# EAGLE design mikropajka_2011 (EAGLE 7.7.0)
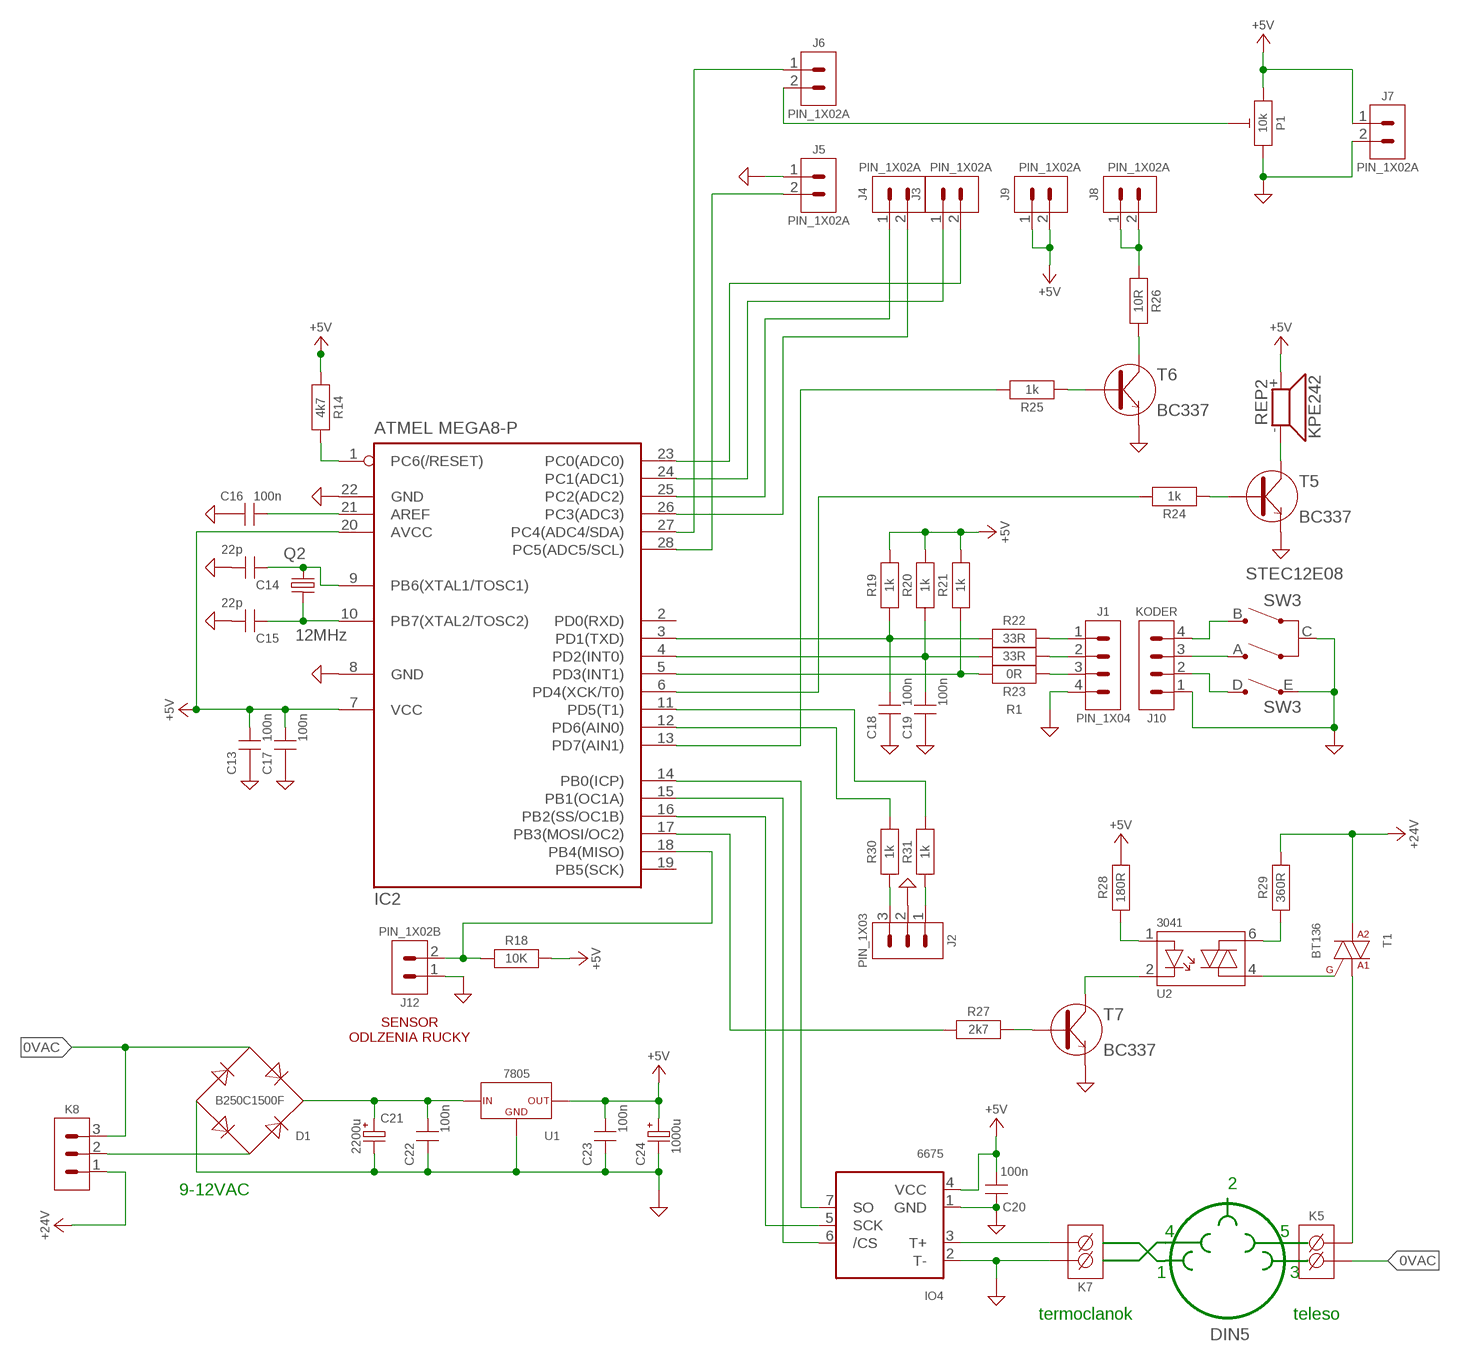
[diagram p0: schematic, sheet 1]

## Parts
C13  100n  KERAMICKYA  [CK_5.08/A]
C14  22p  KERAMICKYB  [CK_5.08/B]
C15  22p  KERAMICKYB  [CK_5.08/B]
C16  100n  KERAMICKYA  [CK_5.08/A]
C17  100n  KERAMICKYA  [CK_5.08/A]
C18  100n  KERAMICKYA  [CK_5.08/A]
C19  100n  KERAMICKYA  [CK_5.08/A]
C20  100n  KERAMICKYA  [CK_5.08/A]
C21  2200u  ELEKTROLYTICKYD  [CE_7.5/A]
C22  100n  KERAMICKYA  [CK_5.08/A]
C23  100n  KERAMICKYA  [CK_5.08/A]
C24  1000u  ELEKTROLYTICKYC  [CE_5.08/B]
D1  B250C1500F  USMERNOVACI_MOSTIKA  [D.USMERNOVAC/GULATY]
IC2  ATMEL MEGA8-P  MEGA8-P  [DIL28-3]
IO4  6675  MAX6675  [SO08]
J1  PIN_1X04  [1X04]
J2  PIN_1X03  [1X03]
J3  PIN_1X02A  [1X02/A]
J4  PIN_1X02A  [1X02/A]
J5  PIN_1X02A  [1X02/A]
J6  PIN_1X02A  [1X02/A]
J7  PIN_1X02A  [1X02/A]
J8  PIN_1X02A  [1X02/A]
J9  PIN_1X02A  [1X02/A]
J10  KODER  PIN_1X04  [1X04]
J12  PIN_1X02B  [1X02/B]
K5  AKZ692/2  [AKZ692/2]
K7  AKZ692/2  [AKZ692/2]
K8  PSH02/3A  [PSH02/3A]
P1  10k  TRIMERE  [CA6]
Q2  12MHz  XTAL  [HC-49/U]
R1  0R  REZISTORA  [0207_10]
R14  4k7  REZISTORA  [0207_10]
R18  10K  REZISTOR  [0207_STOJATY]
R19  1k  REZISTORA  [0207_10]
R20  1k  REZISTORA  [0207_10]
R21  1k  REZISTORA  [0207_10]
R22  33R  REZISTORA  [0207_10]
R23  33R  REZISTORA  [0207_10]
R24  1k  REZISTORA  [0207_10]
R25  1k  REZISTORA  [0207_10]
R26  10R  REZISTORA  [0207_10]
R27  2k7  REZISTORA  [0207_10]
R28  180R  REZISTORA  [0207_10]
R29  360R  REZISTORA  [0207_10]
R30  1k  REZISTORA  [0207_10]
R31  1k  REZISTORA  [0207_10]
REP2  KPE242  [KPE242]
SW3  STEC12E08  KODER_ROTACNIEC12  [EC12]
T1  BT136  [TO220]
T5  BC337  [TO-92]
T6  BC337  [TO-92]
T7  BC337  [TO-92]
U1  7805  78..  [TO220]
U2  3041  MOC3041  [DIL6]

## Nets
0VAC: D1.AC+ K5.1 K8.3
24VAC: K8.1 R29.2 T1.2(A2) ; supply symbol labelled +24V
+5V: C13.C1 C17.C1 C20.C1 C23.C1 C24.C+ IC2.7(VCC) IC2.20(AVCC) IO4.4(VCC) J7.1 J9.1 J9.2 P1.3 R14.1 R18.2 R19.2 R20.2 R21.2 R28.2 REP2.+ U1.P3(OUT)
GND: C13.C2 C14.C1 C15.C1 C16.C2 C17.C2 C18.C2 C19.C2 C20.C2 C21.C- C22.C2 C23.C2 C24.C- D1.DC- IC2.8(GND) IC2.22(GND) IO4.1(GND) IO4.2(T-) J1.4 J2.2 J5.1 J7.2 J10.1 J12.1 K7.2 P1.1 SW3.C(A:C) SW3.E(B:E) T5.3(E) T6.3(E) T7.3(E) U1.P2(GND)
N$1: IC2.27(PC4(ADC4/SDA)) J6.1
N$2: J6.2 P1.2
N$3: J1.3 R1.1
N$4: C15.C2 IC2.10(PB7(XTAL2/TOSC2)) Q2.1
N$11: J8.1 J8.2 R26.1
N$41: C14.C2 IC2.9(PB6(XTAL1/TOSC1)) Q2.2
N$42: C16.C1 IC2.21(AREF)
N$43: IC2.1(PC6(/RESET)) R14.2
N$45: IC2.18(PB4(MISO)) J12.2 R18.1
N$48: R26.2 T6.1(C)
N$49: C18.C1 IC2.3(PD1(TXD)) R19.1 R22.2
N$50: C19.C1 IC2.4(PD2(INT0)) R20.1 R23.2
N$51: IC2.5(PD3(INT1)) R1.2 R21.1
N$52: J1.1 R22.1
N$53: J1.2 R23.1
N$54: IC2.13(PD7(AIN1)) R25.2
N$55: R24.1 T5.2(B)
N$56: IC2.6(PD4(XCK/T0)) R24.2
N$57: REP2.- T5.1(C)
N$58: IC2.17(PB3(MOSI/OC2)) R27.1
N$59: R25.1 T6.2(B)
N$60: R27.2 T7.2(B)
N$61: T7.1(C) U2.2
N$62: R28.1 U2.1
N$63: R29.1 U2.6
N$64: T1.3(G) U2.4
N$66: K5.2 T1.1(A1)
N$68: J2.3 R30.1
N$69: J2.1 R31.1
N$70: IC2.12(PD6(AIN0)) R30.2
N$71: IC2.11(PD5(T1)) R31.2
N$73: IO4.3(T+) K7.1
N$74: J10.4 SW3.B(A:B)
N$75: J10.3 SW3.A(A:A)
N$76: IC2.14(PB0(ICP)) IO4.7(SO)
N$77: IC2.15(PB1(OC1A)) IO4.6(/CS)
N$78: IC2.16(PB2(SS/OC1B)) IO4.5(SCK)
N$79: J10.2 SW3.D(B:D)
N$85: IC2.28(PC5(ADC5/SCL)) J5.2
N$87: IC2.23(PC0(ADC0)) J3.2
N$88: IC2.24(PC1(ADC1)) J3.1
N$89: IC2.25(PC2(ADC2)) J4.1
N$90: IC2.26(PC3(ADC3)) J4.2
N$91: C21.C+ C22.C1 D1.DC+ U1.P1(IN)
N$94: D1.AC- K8.2
Unconnected: IC2.2(PD0(RXD)) IC2.19(PB5(SCK))

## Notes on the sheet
- SENSOR
  ODLZENIA RUCKY
- 9-12VAC | 2
- 4 | 5
- 1 | 3
- termoclanok | teleso
- DIN5

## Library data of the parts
C13-C20 C22 C23 = Kondenzatory:KERAMICKY: Keramicky kondenzator
C21 C24 = Kondenzatory:ELEKTROLYTICKY: Elektrolyticky kondenzator
D1 = Diody:USMERNOVACI_MOSTIK: Usmeronovaci mostik
IC2 = atmel:MEGA8-P: MICROCONTROLLER 8 Kbytes FLASH, 1 kbytes SRAM, 512 bytes EEPROM, USART, 4-channel 10 bit ADC, 2-channel 8 bit ADC Pin compatible with Atmega48, ATMega88, ATMega168 Source: avr.lbr; OC_FARNELL: unknown; OC_NEWARK: unknown
IO4 = #PaJa_31:MAX6675: Cold Junction compensated K-Thermocouple to digital converter (0°C to + 1024°C)
J1 J10 = Pin:PIN_1X04: PIN_1x04
J2 = Pin:PIN_1X03: PIN_1x03
J3-J9 J12 = Pin:PIN_1X02: PIN_1x02
K5 K7 = Konektory:AKZ692/2: Svorkovnica 2 PIN
K8 = Konektory:PSH02/3: Konektor molex 3 PIN
P1 = Rezistory:TRIMER: Trimer
Q2 = Rozne:XTAL: Krystal
R1 R14 R18-R31 = Rezistory:REZISTOR: Rezistor 0207
REP2 = #PaJa_31:KPE242: Piezo-sirenka - 70dB - 3V az 16V
SW3 = #PaJa_22:KODER_ROTACNI: Rotacni koder se spinacem v hrideli www.tme.cz
T1 = Triak:BT136: BT136
T5-T7 = #PaJa_30:BC337: Tranzistor NPN - Univerzalni NF - Ic=0,5A
U1 = Stabilizatory:78..: Linearny stabilizator napatia 78.. (pozitivny)
U2 = Optotriak:MOC3041: Optotriak MOC3041

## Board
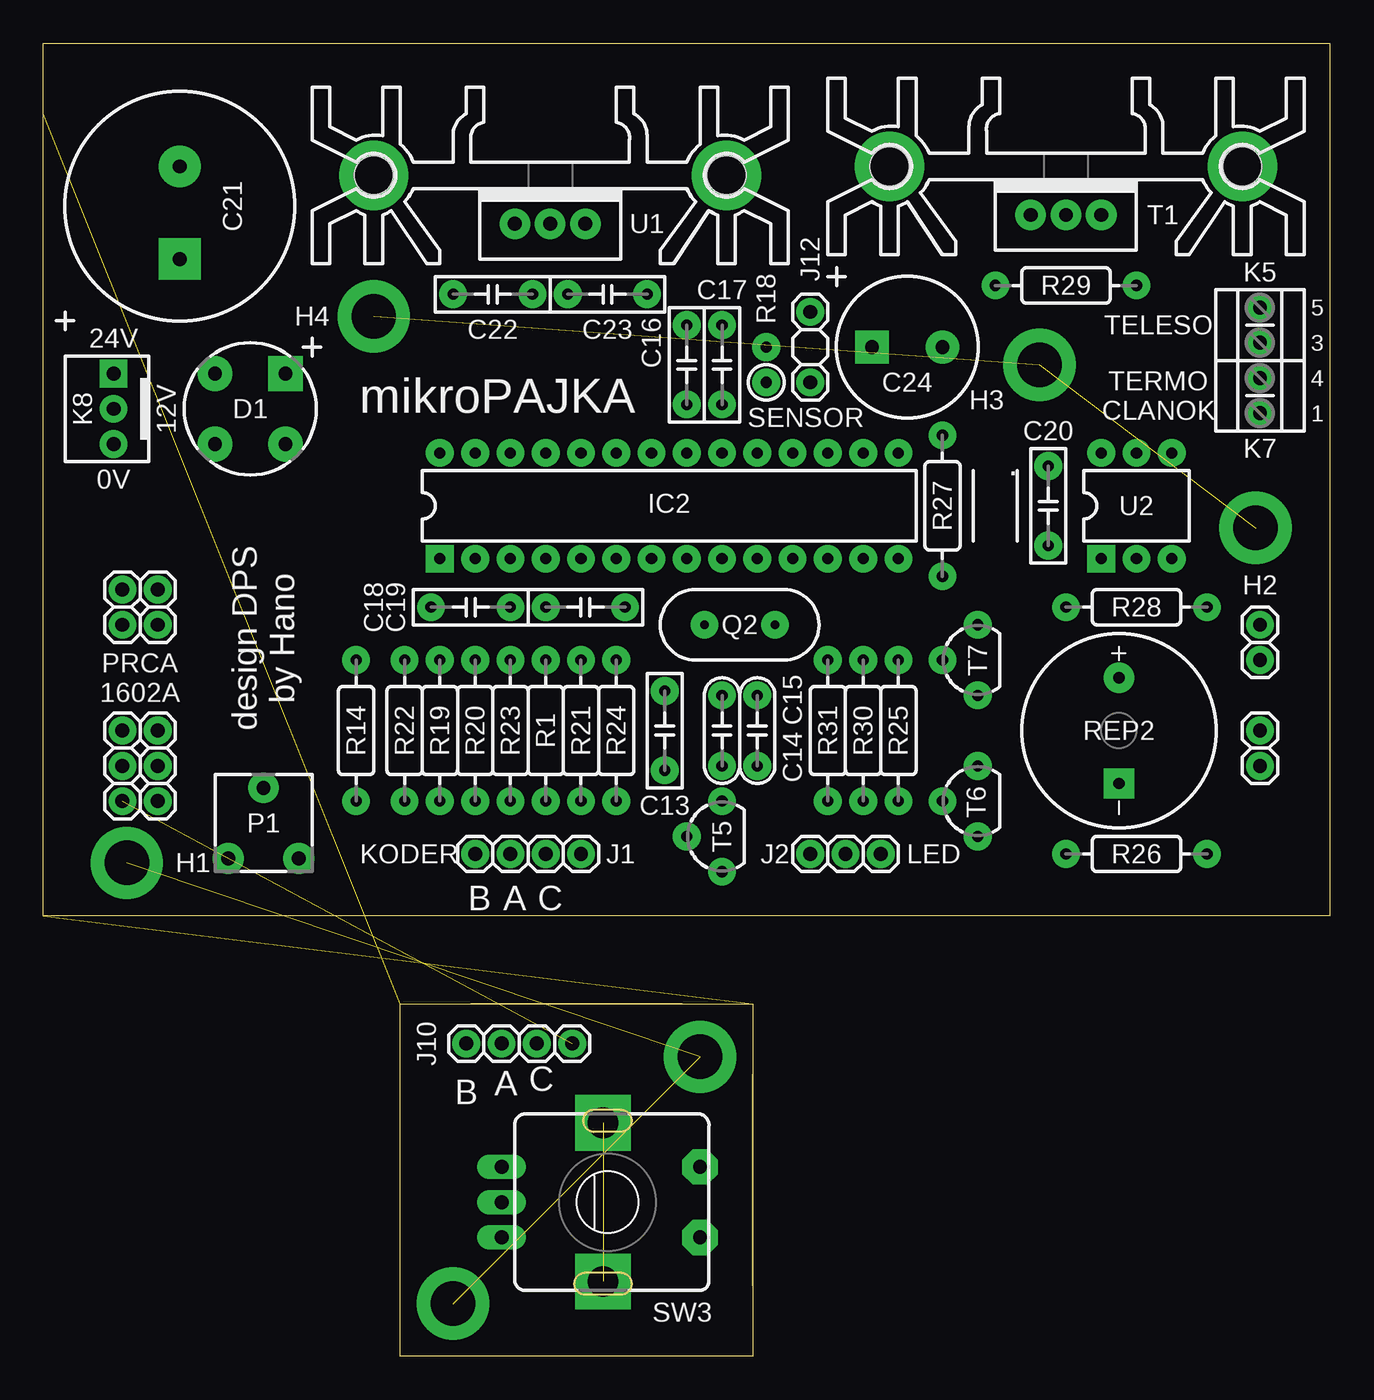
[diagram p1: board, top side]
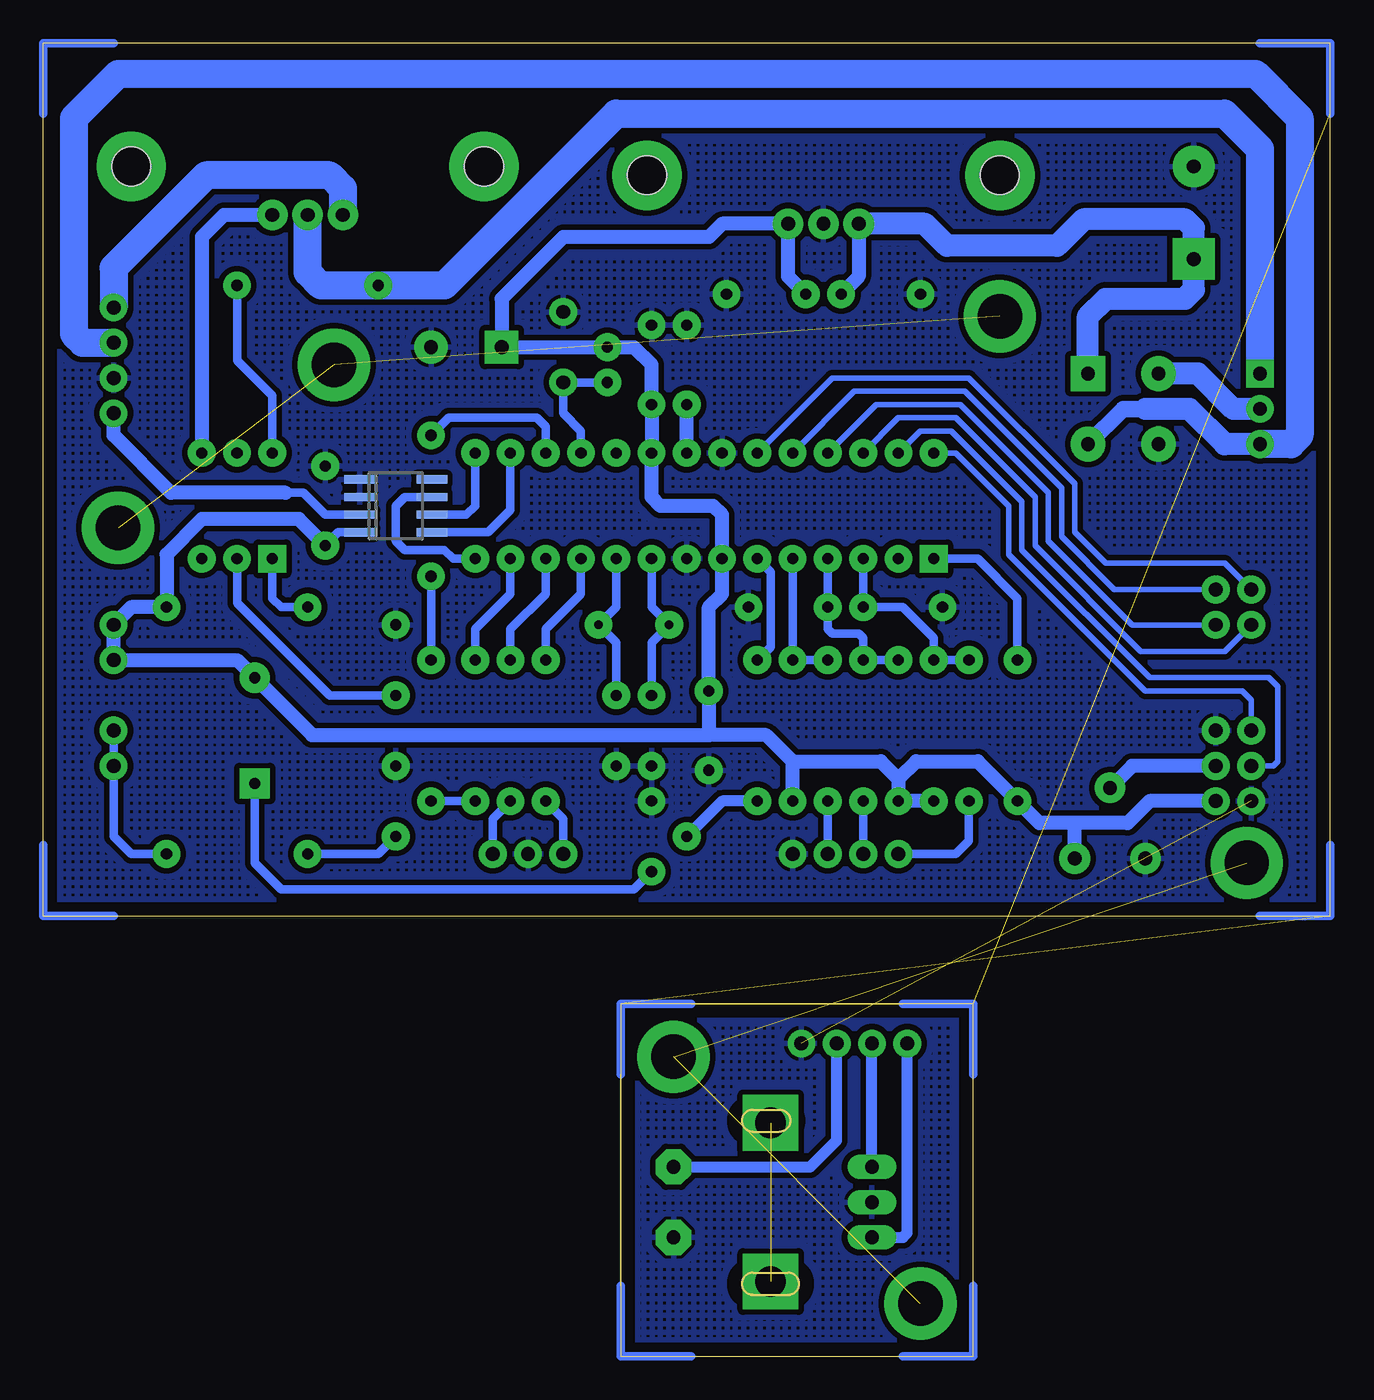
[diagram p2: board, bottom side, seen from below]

Size 92.71 x 94.62 mm. Coordinates in mm from the lower left corner, seen from the top.
Outline: 0,31.75 0,94.62 92.71,94.62 92.71,31.75 0,31.75
Outline: 25.72,25.4 51.12,25.4 51.12,0 25.72,0 25.72,25.4
Copper layers (1*16): Top 0.035mm / dielectric 1.5mm / Bottom 0.035mm
Design rules "default *": minimum track width 10mil, minimum drill 24mil, track to track 8mil, track to pad 8mil, pad to pad 8mil, via to via 8mil, smd to smd 8mil, copper to edge 40mil, drill to drill 8mil, minimum pad ring 10mil, minimum via ring 8mil, stop-mask expansion 4mil, vias tented up to drill 0mil, thermal gap 10mil

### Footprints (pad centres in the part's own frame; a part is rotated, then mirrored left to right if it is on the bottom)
CK_5.08/A = drill 0.8 pad 2: C1 -2.857,0; C2 2.857,0
CK_5.08/B = drill 0.8 pad 2: C1 -2.54,0; C2 2.54,0
CE_7.5/A = drill 1 pad 3 square: C+ -3.81,0 | drill 1 pad 3: C- 2.857,0
CE_5.08/B = drill 1 pad 2.4 square: C+ -2.54,0 | drill 1 pad 2.4: C- 2.54,0
D.USMERNOVAC/GULATY = drill 1 pad 2.5: AC+ 2.54,2.54; AC- -2.54,-2.54; DC- 2.54,-2.54 | drill 1 pad 2.5 square: DC+ -2.54,2.54
DIL28-3 = drill 0.8 pad 2 square: 1 -16.51,-3.81 | drill 0.8 pad 2: 2 -13.97,-3.81; 3 -11.43,-3.81; 4 -8.89,-3.81; 5 -6.35,-3.81; 6 -3.81,-3.81; 7 -1.27,-3.81; 8 1.27,-3.81; 9 3.81,-3.81; 10 6.35,-3.81; 11 8.89,-3.81; 12 11.43,-3.81; 13 13.97,-3.81; 14 16.51,-3.81; 15 16.51,3.81; 16 13.97,3.81; 17 11.43,3.81; 18 8.89,3.81; 19 6.35,3.81; 20 3.81,3.81; 21 1.27,3.81; 22 -1.27,3.81; 23 -3.81,3.81; 24 -6.35,3.81; 25 -8.89,3.81; 26 -11.43,3.81; 27 -13.97,3.81; 28 -16.51,3.81
SO08 = smd 0.6 x 2.2: 1 -1.905,-2.6; 2 -0.635,-2.6; 3 0.635,-2.6; 4 1.905,-2.6; 5 1.905,2.6; 6 0.635,2.6; 7 -0.635,2.6; 8 -1.905,2.6
1X04 = drill 1 pad 2: 1 -3.81,0; 2 -1.27,0; 3 1.27,0; 4 3.81,0
1X03 = drill 1 pad 2: 1 -2.54,0; 2 0,0; 3 2.54,0
1X02/A = drill 1 pad 2: 1 -1.27,0; 2 1.27,0
1X02/B = drill 1 pad 2: 1 -2.54,0; 2 2.54,0
AKZ692/2 = drill 1 pad 2: 1 -1.27,0; 2 1.27,0
PSH02/3A = drill 1 pad 2 square: 1 -2.54,0 | drill 1 pad 2: 2 0,0; 3 2.54,0
CA6 = drill 1 pad 2.2: 1 -2.54,-2.54; 2 0,2.54; 3 2.54,-2.54
HC-49/U = drill 0.6 pad 2: 1 -2.54,0; 2 2.54,0
0207_10 = drill 0.8 pad 2: 1 -5.08,0; 2 5.08,0
0207_STOJATY = drill 0.8 pad 2: 1 -1.27,0; 2 1.27,0
KPE242 = drill 0.813 pad 2.184: + -3.81,0 | drill 0.813 pad 2.184 square: - 3.81,0
EC12 = drill 1 pad 1.778 long: A -2.54,-7.62; B 2.54,-7.62; C 0,-7.62 | drill 1 pad 2.54 octagon: D -2.54,6.668; E 2.54,6.668
TO220 = drill 1 pad 2.2: 1 -2.54,0; 2 0,0; 3 2.54,0
TO-92 = drill 0.8 pad 2: 1 0,2.54; 2 2.54,0; 3 0,-2.54
TO220' = drill 1 pad 2.2: P1 -2.54,0; P2 0,0; P3 2.54,0
DIL6 = drill 0.8 pad 2 square: 1 -2.54,-3.81 | drill 0.8 pad 2: 2 0,-3.81; 3 2.54,-3.81; 4 2.54,3.81; 5 0,3.81; 6 -2.54,3.81
CH_HS-135A = hole 2.8: -12.7,0; 12.7,0

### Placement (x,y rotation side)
C13  44.77,45.09 270 top
C14  48.89,45.09 90 top
C15  51.44,45.09 90 top
C16  46.35,71.44 90 top
C17  48.89,71.44 90 top
C18  30.8,53.98 180 top
C19  39.05,53.98 0 top
C20  72.39,61.28 90 top
C21  9.84,82.87 90 top
C22  32.38,76.52 180 top
C23  40.64,76.52 0 top
C24  62.23,72.71 0 top
D1  14.92,68.26 270 top
IC2  45.09,61.28 0 top
IO4  67.31,61.28 270 bottom
J1  34.92,36.2 0 top
J2  57.78,36.2 0 top
J3  6.99,55.25 180 top
J4  6.99,52.7 180 top
J5  6.99,45.09 180 top
J6  6.99,42.55 0 top
J7  6.99,40.01 180 top
J8  87.63,43.81 90 top
J9  87.63,51.44 90 top
J10  34.29,22.54 180 top
J12  55.24,72.71 270 top
K5  87.63,74.3 90 top
K7  87.63,69.22 90 top
K8  5.08,68.26 270 top
P1  15.88,38.42 0 top
Q2  50.16,52.7 180 top
R1  36.2,45.09 90 top
R14  22.54,45.09 90 top
R18  52.07,71.44 90 top
R19  28.57,45.09 270 top
R20  31.12,45.09 270 top
R21  38.73,45.09 270 top
R22  26.04,45.09 90 top
R23  33.66,45.09 90 top
R24  41.27,45.09 90 top
R25  61.59,45.09 90 top
R26  78.74,36.2 180 top
R27  64.77,61.28 270 top
R28  78.74,53.98 0 top
R29  73.66,77.15 180 top
R30  59.05,45.09 90 top
R31  56.52,45.09 90 top
REP2  77.47,45.09 270 top
SW3  40.64,11.11 270 top
T1  73.66,82.23 0 top
T5  48.89,37.47 180 top
T6  67.31,40.01 180 top
T7  67.31,50.16 180 top
U1  7805  [TO220']  36.51,81.6 0 top
U2  78.74,61.28 0 top
U$34  [CH_HS-135A]  36.51,85.09 0 top
U$35  [CH_HS-135A]  73.66,85.72 0 top

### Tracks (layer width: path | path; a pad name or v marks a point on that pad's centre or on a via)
0VAC
  Bottom 1.2: D1.AC+ 14.92,68.26 13.33,68.26
  Bottom 1.6: K8.3 7.62,65.72 10.16,68.26 13.33,68.26
  Bottom 2: K8.3 2.86,65.72 2.22,66.36 2.22,89.22 5.4,92.39 87.31,92.39 90.49,89.22 90.49,73.66 89.85,73.03 K5.1
24VAC
  Bottom 2: T1.2 73.66,78.1 72.71,77.15 R29.2 63.82,77.15 51.44,89.53 7.62,89.53 5.08,87 K8.1
+5V
  Bottom 0.6: IO4.4 71.44,59.37 C20.C1
  Bottom 1: C23.C1 39.05,77.79 U1.P3 43.81,81.6 44.77,80.65 55.24,80.65 59.69,76.2 C24.C+ R18.2 50.16,72.71 48.89,71.44 C17.C1 IC2.20 48.89,61.91 48.26,61.28 44.45,61.28 43.81,60.64 IC2.7 43.81,54.93 44.77,53.98 C13.C1 44.77,44.77 | C20.C1 74.3,60.33 81.28,60.33 83.82,57.78 R28.2 86.36,53.98 J9.2 J9.1 78.74,50.16 REP2.+ 73.34,44.77 44.77,44.77 | R21.2 38.74,42.86 | R19.2 R20.2 31.12,41.59 | 38.74,42.86 32.38,42.86 31.12,41.59 | 31.12,41.59 29.84,42.86 25.4,42.86 R14.1 20.95,38.42 18.41,38.42 | J7.1 13.02,40.01 14.6,38.42 18.41,38.42 | P1.3 18.41,38.42 | 38.74,42.86 40.64,44.77 44.77,44.77
GND  (1 unrouted)
  pour Bottom (isolate 0.4, hatched): 0,94.62 92.71,94.62 92.71,31.75 0,31.75
  pour Bottom (isolate 0.4, hatched): 25.72,25.4 51.12,25.4 51.12,0 25.72,0
N$1
  Bottom 0.4: IC2.27 29.53,66.67 27.31,66.67 22.22,61.59 22.22,58.1 13.02,48.89 4.44,48.89 3.81,48.26 3.81,42.86 4.13,42.55 J6.1
N$2
  Bottom 1: J6.2 14.29,42.55 P1.2
N$3
  Bottom 0.6: R1.1 J1.3
N$4
  Bottom 0.6: IC2.10 51.44,53.98 Q2.1 51.44,51.44 C15.C2
N$5  (via drill 2.8 pad 5)
  other vias: 23.81,85.09
N$6  (via drill 2.8 pad 5)
  other vias: 49.21,85.09
N$7  (via drill 2.8 pad 5)
  other vias: 60.96,85.72
N$8  (via drill 2.8 pad 5)
  other vias: 86.36,85.72
N$9  (via drill 3.2 pad 5.2)  (2 unrouted)
  other vias: 6.03,35.56 47.31,21.59 29.53,3.81
N$10  (via drill 3.2 pad 5.2)  (2 unrouted)
  other vias: 87.31,59.69 71.75,71.44 23.81,74.93
N$11
  Bottom 0.6: R26.1 86.36,36.2 87.63,37.47 J8.1 J8.2
N$12  (via drill 2.2 pad 4)  (1 unrouted)
  other vias: 40.32,16.83 40.32,5.4
N$13  (7 unrouted)
  Bottom 0.6: 0,89.53 0,94.62 5.08,94.62 | 87.63,94.62 92.71,94.62 92.71,89.53 | 87.63,31.75 92.71,31.75 92.71,36.83 | 0,36.83 0,31.75 5.08,31.75 | 51.12,20.32 51.12,25.4 46.04,25.4 | 46.04,0 51.12,0 51.12,5.08 | 30.8,0 25.72,0 25.72,5.08 | 25.72,20.32 25.72,25.4 30.8,25.4
N$41
  Bottom 0.6: IC2.9 48.89,53.98 Q2.2 48.89,51.44 C14.C2
N$42
  Bottom 1: IC2.21 C16.C1
N$43
  Bottom 0.6: IC2.1 25.4,57.47 22.54,54.61 R14.2
N$45
  Bottom 0.6: IC2.18 53.98,66.67 55.24,67.94 J12.2 R18.1
N$48
  Bottom 0.6: R26.2 68.58,36.2 T6.1
N$49
  Bottom 0.6: R22.2 R19.1 28.57,51.75 30.8,53.98 C18.C1 IC2.3
N$50
  Bottom 0.6: R20.1 R23.2 33.66,51.75 33.97,52.07 35.88,52.07 36.2,52.39 C19.C1 IC2.4
N$51
  Bottom 0.6: IC2.5 R21.1 R1.2
N$52
  Bottom 0.6: J1.1 26.99,36.2 26.04,37.15 R22.1
N$53
  Bottom 0.6: J1.2 R23.1
N$54
  Bottom 0.6: IC2.13 59.06,54.93 61.59,52.39 R25.2
N$55
  Bottom 0.8: R24.1 43.81,40.01 T5.2
N$56
  Bottom 0.6: R24.2 40.32,51.12 40.32,56.52 IC2.6
N$57
  Bottom 0.6: T5.1 50.16,33.66 75.56,33.66 77.47,35.56 REP2.-
N$58
  Bottom 0.6: R27.1 63.5,67.63 57.15,67.63 56.52,66.99 IC2.17
N$59
  Bottom 0.6: R25.1 T6.2
N$60
  Bottom 0.6: R27.2 T7.2
N$61
  Bottom 0.6: T7.1 72.07,47.62 78.74,54.29 U2.2
N$62
  Bottom 0.6: U2.1 76.2,54.61 75.56,53.98 R28.1
N$63
  Bottom 0.6: R29.1 78.74,71.75 76.2,69.22 U2.6
N$64
  Bottom 1: T1.3 79.69,82.23 81.28,80.65 U2.4
N$66
  Bottom 2: T1.1 71.12,84.14 72.07,85.09 80.96,85.09 87.63,78.42 K5.2
N$68
  Bottom 0.6: J2.3 60.33,38.73 R30.1
N$69
  Bottom 0.6: J2.1 55.24,38.73 R31.1
N$70
  Bottom 0.6: IC2.12 56.52,54.93 59.06,52.39 R30.2
N$71
  Bottom 0.6: IC2.11 53.98,54.93 56.52,52.39 R31.2
N$73
  Bottom 0.6: IO4.3 72.39,60.64 73.98,62.23 75.25,62.23
  Bottom 1: K7.1 87.63,66.36 83.5,62.23 75.25,62.23
N$74
  Bottom 0.8: SW3.B 30.8,8.57 30.48,8.89 J10.4
N$75
  Bottom 0.8: SW3.A J10.3
N$76
  Bottom 0.6: IC2.14 63.18,57.47 63.82,58.1 66.67,58.1 67.31,58.74 67.31,61.28 66.67,61.91 IO4.7
N$77
  Bottom 0.6: IC2.15 61.59,61.28 62.23,60.64 IO4.6
N$78
  Bottom 0.6: IO4.5 60.64,59.37 59.06,60.96 IC2.16
N$79
  Bottom 0.8: SW3.D 37.46,13.65 35.56,15.56 J10.2
N$85
  Bottom 0.4: IC2.28 26.99,65.09 23.18,61.28 23.18,57.78 13.33,47.94 6.35,47.94 5.72,47.31 J5.2
N$87
  Bottom 0.4: IC2.23 35.88,70.48 26.04,70.48 18.41,62.86 18.41,59.37 16.19,57.15 7.62,57.15 J3.2
N$88
  Bottom 0.4: IC2.24 34.29,69.53 26.35,69.53 19.37,62.55 19.37,59.05 15.56,55.25 J3.1
N$89
  Bottom 0.4: IC2.25 32.7,68.58 26.67,68.58 20.32,62.23 20.32,58.74 14.29,52.7 J4.1
N$90
  Bottom 0.4: IC2.26 31.12,67.63 26.99,67.63 21.27,61.91 21.27,58.42 13.65,50.8 7.62,50.8 J4.2
N$91
  Bottom 1: C22.C1 33.97,77.79 U1.P1
  Bottom 1.6: D1.DC+ 17.46,74.93 16.19,76.2 10.48,76.2 9.84,76.84 C21.C+ 9.84,81.28 10.48,81.91 17.78,81.91 19.68,80.01 27.62,80.01 29.21,81.6 U1.P1
N$94
  Bottom 1.6: K8.2 6.99,68.26 9.52,70.8 D1.AC-

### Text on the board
tPlace: 5 | H4 | TELESO | 24V | 3 | 4 | 12V | mikroPAJKA | H3 | TERMO / CLANOK | SENSOR | 1 | . | 0V | H2 | design DPS / by Hano | PRCA / 1602A | H1 | KODER | LED | B | A | C | A | C | B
